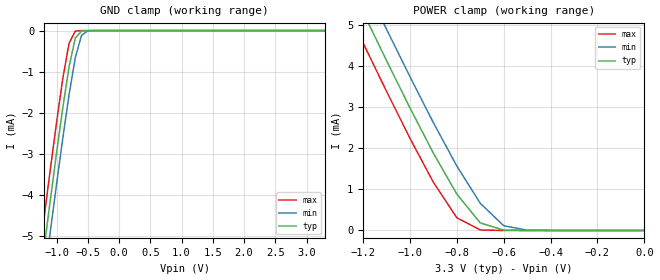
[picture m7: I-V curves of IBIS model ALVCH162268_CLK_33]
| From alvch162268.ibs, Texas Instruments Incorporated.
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|************* ALVCH162268 INPUT (3.3 V) MODEL**************
[Model]   ALVCH162268_CLK_33
Model_type  Input
Polarity   Non-Inverting
Vinl = 0.8V
Vinh = 2.0V
| variable   typ   min   max
C_comp   2.15pF   NA   NA
[Temperature Range]   50   100   0
[Voltage range]   3.3   3   3.6
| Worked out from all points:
|   GND clamp passes 1 mA (typ) near -0.81 V on its own axis
|   POWER clamp passes 1 mA (typ) near -0.81 V on its own axis
|Process range|   weak   strong
[GND Clamp]
|   50C:3.3V:   100C:3V:weak   0C:3.6V:strong
|   Voltage   I(typ)   I(min)   I(max)
-3.3V     -31.29mA   -32.01mA   -30.61mA
-1.3V     -6.503mA   -7.266mA   -5.756mA
-1.2V     -5.308mA   -6.072mA   -4.559mA
-1.1V     -4.131mA   -4.895mA   -3.383mA
-1V       -2.981mA   -3.739mA   -2.24mA
-900mV    -1.879mA   -2.62mA    -1.171mA
-800mV    -884.1uA   -1.566mA   -309.4uA
-700mV    -183.9uA   -659.5uA   -12.88uA
-600mV    -8.941uA   -116.2uA   -211.8nA
-500mV    -274.5nA   -7.235uA   -3.352nA
3.3V      6.336pA    16.94nA    5.74pA
[POWER Clamp]
|   50C:3.3V:   100C:3V:weak   0C:3.6V:strong
|   Voltage   I(typ)   I(min)   I(max)
-3.3V     31.29mA    32.01mA    30.61mA
-1.3V     6.503mA    7.266mA    5.756mA
-1.2V     5.308mA    6.072mA    4.559mA
-1.1V     4.131mA    4.895mA    3.382mA
-1V       2.98mA     3.739mA    2.24mA
-900mV    1.879mA    2.62mA     1.171mA
-800mV    884.1uA    1.566mA    309.4uA
-700mV    183.9uA    659.4uA    12.88uA
-600mV    8.941uA    116.1uA    211.8nA
-500mV    274.5nA    7.235uA    3.352nA
0V        6.336pA    7.803pA    6.787pA
